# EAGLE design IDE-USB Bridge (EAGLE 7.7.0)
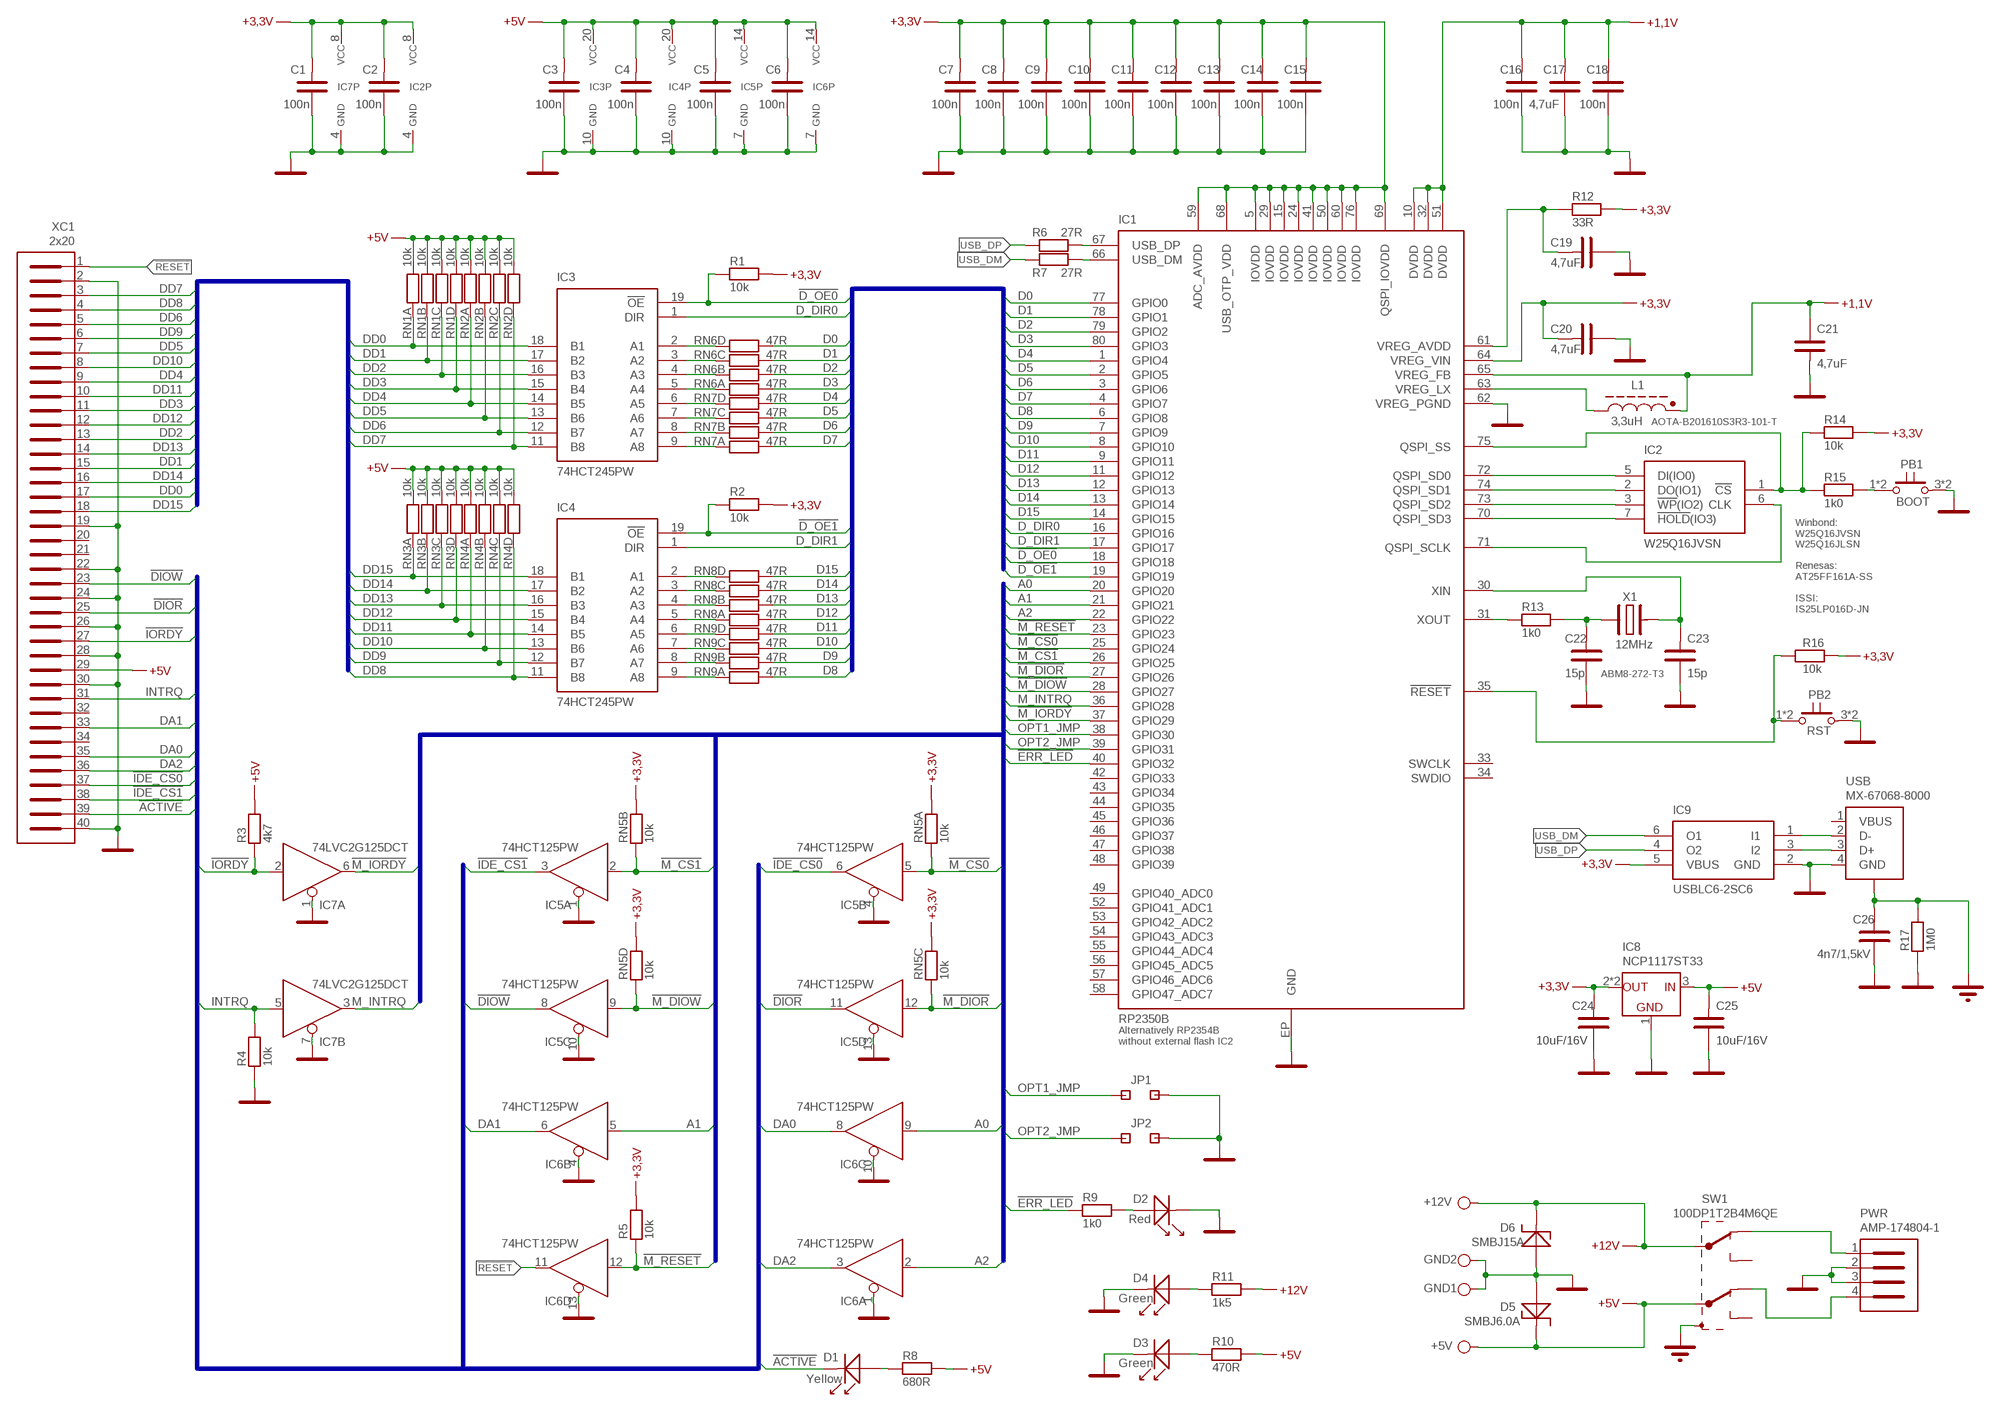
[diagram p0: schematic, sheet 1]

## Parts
+5V  +5V  PAJ_B_16  [P_BOD_16]
+12V  +12V  PAJ_B_16  [P_BOD_16]
C1  100n  CK-SMD-0603  [CK-0603]
C2  100n  CK-SMD-0603  [CK-0603]
C3  100n  CK-SMD-0603  [CK-0603]
C4  100n  CK-SMD-0603  [CK-0603]
C5  100n  CK-SMD-0603  [CK-0603]
C6  100n  CK-SMD-0603  [CK-0603]
C7  100n  CK-SMD-0603  [CK-0603]
C8  100n  CK-SMD-0603  [CK-0603]
C9  100n  CK-SMD-0603  [CK-0603]
C10  100n  CK-SMD-0603  [CK-0603]
C11  100n  CK-SMD-0603  [CK-0603]
C12  100n  CK-SMD-0603  [CK-0603]
C13  100n  CK-SMD-0603  [CK-0603]
C14  100n  CK-SMD-0603  [CK-0603]
C15  100n  CK-SMD-0603  [CK-0603]
C16  100n  CK-SMD-0603  [CK-0603]
C17  4,7uF  CK-SMD-0603  [CK-0603]
C18  100n  CK-SMD-0603  [CK-0603]
C19  4,7uF  CK-SMD-0603  [CK-0603]
C20  4,7uF  CK-SMD-0603  [CK-0603]
C21  4,7uF  CK-SMD-0603  [CK-0603]
C22  15p  CK-SMD-0805  [CK-0805]
C23  15p  CK-SMD-0805  [CK-0805]
C24  10uF/16V  CK-SMD-1206  [CK-1206]
C25  10uF/16V  CK-SMD-1206  [CK-1206]
C26  4n7/1,5kV  CK-SMD-1206  [CK-1206]
D1  Yellow  LED-1206  [LED1206K]
D2  Red  LED-1206  [LED1206K]
D3  Green  LED-1206  [LED1206K]
D4  Green  LED-1206  [LED1206K]
D5  SMBJ6.0A  600W-USM  [DO-214AA]
D6  SMBJ15A  600W-USM  [DO-214AA]
GND1  GND  PAJ_B_16  [P_BOD_16]
GND2  GND  PAJ_B_16  [P_BOD_16]
IC1  RP2350B  RP2350  [QFN80]
IC2  W25Q16JVSN  W25Q16-SN  [SO8]
IC3  74HCT245PW  74245-PW  [TSSOP20]
IC4  74HCT245PW  74245-PW  [TSSOP20]
IC5  74HCT125PW  74125-DT  [TSSOP14]
IC6  74HCT125PW  74125-DT  [TSSOP14]
IC7  74LVC2G125DCT  742G125-DP  [SSOP8]
IC8  NCP1117ST33  LDL1117  [SOT223]
IC9  USBLC6-2SC6  [SOT23-6]
JP1  JMP2-1  [JMP2-1]
JP2  JMP2-1  [JMP2-1]
L1  3,3uH  TL-SMD-2016  [TL-2016]
PB1  BOOT  TL-SMD-PTS647  [TL-PTS647]
PB2  RST  TL-SMD-PTS647  [TL-PTS647]
PWR  AMP-174804-1  AMP174804  [AMP174804]
R1  10k  R-SMD-0805  [R-0805]
R2  10k  R-SMD-0805  [R-0805]
R3  4k7  R-SMD-0805  [R-0805]
R4  10k  R-SMD-0805  [R-0805]
R5  10k  R-SMD-0805  [R-0805]
R6  27R  R-SMD-0805  [R-0805]
R7  27R  R-SMD-0805  [R-0805]
R8  680R  R-SMD-1206  [R-1206]
R9  1k0  R-SMD-1206  [R-1206]
R10  470R  R-SMD-1206  [R-1206]
R11  1k5  R-SMD-1206  [R-1206]
R12  33R  R-SMD-0805  [R-0805]
R13  1k0  R-SMD-0805  [R-0805]
R14  10k  R-SMD-0805  [R-0805]
R15  1k0  R-SMD-0805  [R-0805]
R16  10k  R-SMD-0805  [R-0805]
R17  1M0  R-SMD-1206  [R-1206]
RN1  10k  R-NET4SB  [R-NET4SB]
RN2  10k  R-NET4SB  [R-NET4SB]
RN3  10k  R-NET4SB  [R-NET4SB]
RN4  10k  R-NET4SB  [R-NET4SB]
RN5  10k  R-NET4SB  [R-NET4SB]
RN6  47R  R-NET4SB  [R-NET4SB]
RN7  47R  R-NET4SB  [R-NET4SB]
RN8  47R  R-NET4SB  [R-NET4SB]
RN9  47R  R-NET4SB  [R-NET4SB]
SW1  100DP1T2B4M6QE  SW-100DP1T2B  [SW-100DP1T2]
USB  MX-67068-8000  USB-B-B1  [USB-B1]
X1  12MHz  XTAL-SMD-3225  [X-3225-2]
XC1  2x20  25-V2R40-TOP  [25-V2R40T]

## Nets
!ACTIVE: D1.K XC1.39
!D_OE0: IC1.18(GPIO18) IC3.19(!OE) R1.1
!D_OE1: IC1.19(GPIO19) IC4.19(!OE) R2.1
!DIOR: IC5.11(D:O) XC1.25
!DIOW: IC5.8(C:O) XC1.23
!ERR_LED: IC1.40(GPIO32) R9.1
!IDE_CS0: IC5.6(B:O) XC1.37
!IDE_CS1: IC5.3(A:O) XC1.38
!IORDY: IC7.2(A:I) R3.1 XC1.27
!M_CS0: IC1.25(GPIO24) IC5.5(B:I) RN5.1
!M_CS1: IC1.26(GPIO25) IC5.2(A:I) RN5.2
!M_DIOR: IC1.27(GPIO26) IC5.12(D:I) RN5.3
!M_DIOW: IC1.28(GPIO27) IC5.9(C:I) RN5.4
!M_IORDY: IC1.37(GPIO29) IC7.6(A:O)
!M_RESET: IC1.23(GPIO23) IC6.12(D:I) R5.1
!RESET: IC6.11(D:O) XC1.1
+1,1V: C16.2 C17.2 C18.2 C21.1 IC1.10(DVDD10) IC1.32(DVDD32) IC1.51(DVDD51) IC1.65(VREG_FB) L1.2(K)
+3,3V: C1.2 C2.2 C7.2 C8.2 C9.2 C10.2 C11.2 C12.2 C13.2 C14.2 C15.2 C20.2 C24.2 IC1.5(IOVDD5) IC1.15(IOVDD15) IC1.24(IOVDD24) IC1.29(IOVDD29) IC1.41(IOVDD41) IC1.50(IOVDD50) IC1.59(ADC_AVDD) IC1.60(IOVDD60) IC1.64(VREG_VIN) IC1.68(USB_OTP_VDD) IC1.69(QSPI_IOVDD) IC1.76(IOVDD76) IC2.8(VCC) IC7.8(P:VCC) IC8.2(OUT) IC8.4(OUT) IC9.5(VBUS) R1.2 R2.2 R5.2 R12.2 R14.2 R16.2 RN5.A RN5.B RN5.C RN5.D
+5V: +5V.1 C3.2 C4.2 C5.2 C6.2 C25.2 D5.K IC3.20(VCC) IC4.20(VCC) IC5.14(P:VCC) IC6.14(P:VCC) IC8.3(IN) R3.2 R8.2 R10.2 RN1.A RN1.B RN1.C RN1.D RN2.A RN2.B RN2.C RN2.D RN3.A RN3.B RN3.C RN3.D RN4.A RN4.B RN4.C RN4.D SW1.5 XC1.29
+12V: +12V.1 D6.K R11.2 SW1.2
A0: IC1.20(GPIO20) IC6.9(C:I)
A1: IC1.21(GPIO21) IC6.5(B:I)
A2: IC1.22(GPIO22) IC6.2(A:I)
D0: IC1.77(GPIO0) RN6.D
D1: IC1.78(GPIO1) RN6.C
D2: IC1.79(GPIO2) RN6.B
D3: IC1.80(GPIO3) RN6.A
D4: IC1.1(GPIO4) RN7.D
D5: IC1.2(GPIO5) RN7.C
D6: IC1.3(GPIO6) RN7.B
D7: IC1.4(GPIO7) RN7.A
D8: IC1.6(GPIO8) RN9.A
D9: IC1.7(GPIO9) RN9.B
D10: IC1.8(GPIO10) RN9.C
D11: IC1.9(GPIO11) RN9.D
D12: IC1.11(GPIO12) RN8.A
D13: IC1.12(GPIO13) RN8.B
D14: IC1.13(GPIO14) RN8.C
D15: IC1.14(GPIO15) RN8.D
D_DIR0: IC1.16(GPIO16) IC3.1(DIR)
D_DIR1: IC1.17(GPIO17) IC4.1(DIR)
DA0: IC6.8(C:O) XC1.35
DA1: IC6.6(B:O) XC1.33
DA2: IC6.3(A:O) XC1.36
DD0: IC3.18(B1) RN1.1 XC1.17
DD1: IC3.17(B2) RN1.2 XC1.15
DD2: IC3.16(B3) RN1.3 XC1.13
DD3: IC3.15(B4) RN1.4 XC1.11
DD4: IC3.14(B5) RN2.1 XC1.9
DD5: IC3.13(B6) RN2.2 XC1.7
DD6: IC3.12(B7) RN2.3 XC1.5
DD7: IC3.11(B8) RN2.4 XC1.3
DD8: IC4.11(B8) RN4.4 XC1.4
DD9: IC4.12(B7) RN4.3 XC1.6
DD10: IC4.13(B6) RN4.2 XC1.8
DD11: IC4.14(B5) RN4.1 XC1.10
DD12: IC4.15(B4) RN3.4 XC1.12
DD13: IC4.16(B3) RN3.3 XC1.14
DD14: IC4.17(B2) RN3.2 XC1.16
DD15: IC4.18(B1) RN3.1 XC1.18
GND: C1.1 C2.1 C3.1 C4.1 C5.1 C6.1 C7.1 C8.1 C9.1 C10.1 C11.1 C12.1 C13.1 C14.1 C15.1 C16.1 C17.1 C18.1 C19.1 C20.1 C21.2 C22.1 C23.1 C24.1 C25.1 C26.1 D2.K D3.K D4.K D5.A D6.A GND1.1 GND2.1 IC1.62(VREG_PGND) IC1.EP(GND) IC2.4(GND) IC3.10(GND) IC4.10(GND) IC5.1(A:OE) IC5.4(B:OE) IC5.7(P:GND) IC5.10(C:OE) IC5.13(D:OE) IC6.1(A:OE) IC6.4(B:OE) IC6.7(P:GND) IC6.10(C:OE) IC6.13(D:OE) IC7.1(A:OE) IC7.4(P:GND) IC7.7(B:OE) IC8.1(GND) IC9.2(GND) JP1.2 JP2.2 PB1.3 PB1.4 PB2.3 PB2.4 PWR.2 PWR.3 R4.1 R17.1 USB.4(GND) XC1.2 XC1.19 XC1.22 XC1.24 XC1.26 XC1.28 XC1.30 XC1.40
INTRQ: IC7.5(B:I) R4.2 XC1.31
M_INTRQ: IC1.36(GPIO28) IC7.3(B:O)
N$1: IC1.67(USB_DP) R6.2
N$2: IC1.66(USB_DM) R7.2
N$3: IC1.72(QSPI_SD0) IC2.5(DI(IO0))
N$4: IC1.74(QSPI_SD1) IC2.2(DO(IO1))
N$5: IC1.73(QSPI_SD2) IC2.3(!WP!(IO2))
N$6: IC1.70(QSPI_SD3) IC2.7(!HOLD!(IO3))
N$7: IC1.71(QSPI_SCLK) IC2.6(CLK)
N$8: PB1.1 PB1.2 R15.2
N$9: IC1.75(QSPI_SS) IC2.1(!CS) R14.1 R15.1
N$10: IC1.31(XOUT) R13.1
N$11: C22.2 R13.2 X1.1
N$12: C23.2 IC1.30(XIN) X1.3
N$13: IC1.63(VREG_LX) L1.1(Z)
N$14: IC9.1(I1) USB.2(D-)
N$15: C19.2 IC1.61(VREG_AVDD) R12.1
N$16: IC9.3(I2) USB.3(D+)
N$17: IC3.5(A4) RN6.1
N$18: D3.A R10.1
N$19: D2.A R9.2
N$20: D4.A R11.1
N$21: D1.A R8.1
N$24: IC3.4(A3) RN6.2
N$25: IC3.3(A2) RN6.3
N$26: IC3.2(A1) RN6.4
N$27: IC3.9(A8) RN7.1
N$28: IC3.8(A7) RN7.2
N$29: IC3.7(A6) RN7.3
N$30: IC3.6(A5) RN7.4
N$31: IC4.5(A4) RN8.1
N$32: IC4.4(A3) RN8.2
N$33: IC4.3(A2) RN8.3
N$34: IC4.2(A1) RN8.4
N$35: IC4.9(A8) RN9.1
N$36: IC4.8(A7) RN9.2
N$37: IC4.7(A6) RN9.3
N$38: IC4.6(A5) RN9.4
N$39: IC1.35(!RESET) PB2.1 PB2.2 R16.1
N$40: PWR.1 SW1.1
N$41: PWR.4 SW1.4
OPT1_JMP: IC1.38(GPIO30) JP1.1
OPT2_JMP: IC1.39(GPIO31) JP2.1
PE: C26.2 R17.2 SW1.S1(SHLD) SW1.S2(SHLD) USB.S1(S) USB.S2(S)
USB_DM: IC9.6(O1) R7.1
USB_DP: IC9.4(O2) R6.1
Unconnected: IC1.33(SWCLK) IC1.34(SWDIO) IC1.42(GPIO33) IC1.43(GPIO34) IC1.44(GPIO35) IC1.45(GPIO36) IC1.46(GPIO37) IC1.47(GPIO38) IC1.48(GPIO39) IC1.49(GPIO40_ADC0) IC1.52(GPIO41_ADC1) IC1.53(GPIO42_ADC2) IC1.54(GPIO43_ADC3) IC1.55(GPIO44_ADC4) IC1.56(GPIO45_ADC5) IC1.57(GPIO46_ADC6) IC1.58(GPIO47_ADC7) SW1.3 SW1.6 USB.1(VBUS) XC1.20 XC1.21 XC1.32 XC1.34

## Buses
BUS1:D0,D1,D2,D3,D4,D5,D6,D7,D8,D9,D10,D11,D12,D13,D14,D15,D_DIR0,D_DIR1,!D_OE0,!D_OE1
BUS2:DD0,DD1,DD2,DD3,DD4,DD5,DD6,DD7,DD8,DD9,DD10,DD11,DD12,DD13,DD14,DD15
BUS3:!DIOW,!DIOR,!IORDY,INTRQ,DA1,DA0,DA2,!IDE_CS0,!IDE_CS1,!ACTIVE
BUS4:A0,A1,A2,!M_RESET,!M_CS0,!M_CS1,!M_DIOR,!M_DIOW,M_INTRQ,!M_IORDY,OPT1_JMP,OPT2_JMP,!ERR_LED

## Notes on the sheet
- AOTA-B201610S3R3-101-T
- Winbond:
  W25Q16JVSN
  W25Q16JLSN
  
  Renesas:
  AT25FF161A-SS
  
  ISSI:
  IS25LP016D-JN
- ABM8-272-T3
- Alternatively RP2354B
  without external flash IC2

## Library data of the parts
+5V +12V GND1 GND2 = KONSTR:PAJ_B_16
C1-C26 = PASIV:CK-SMD: SMD keramické vícevrstvé kondenzátory
D1-D4 = DISKRET:LED-1206
D5 D6 = DISKRET:600W-USM
IC1 = INTEL:RP2350
IC2 = MEMORY:W25Q16
IC3 IC4 = IC:74245
IC5 IC6 = 74499:74125
IC7 = 74499:742G125
IC8 = IC:LDL1117: LDO, fixed voltage, input 18V max., 1,2A, high PSRR, ST
IC9 = DISKRET:USBLC6-2
JP1 JP2 = KONSTR:JMP2-1
L1 = PASIV:TL-SMD
PB1 PB2 = KONSTR:TL-SMD
PWR = CONNEC:AMP174804
R1-R17 = PASIV:R-SMD: SMD rezistory
RN1-RN9 = PASIV:R-NET4SB
SW1 = KONSTR:SW-100DP1T2B
USB = CONNEC:USB-B
X1 = PASIV:XTAL-SMD
XC1 = CONNEC:25-V2R40

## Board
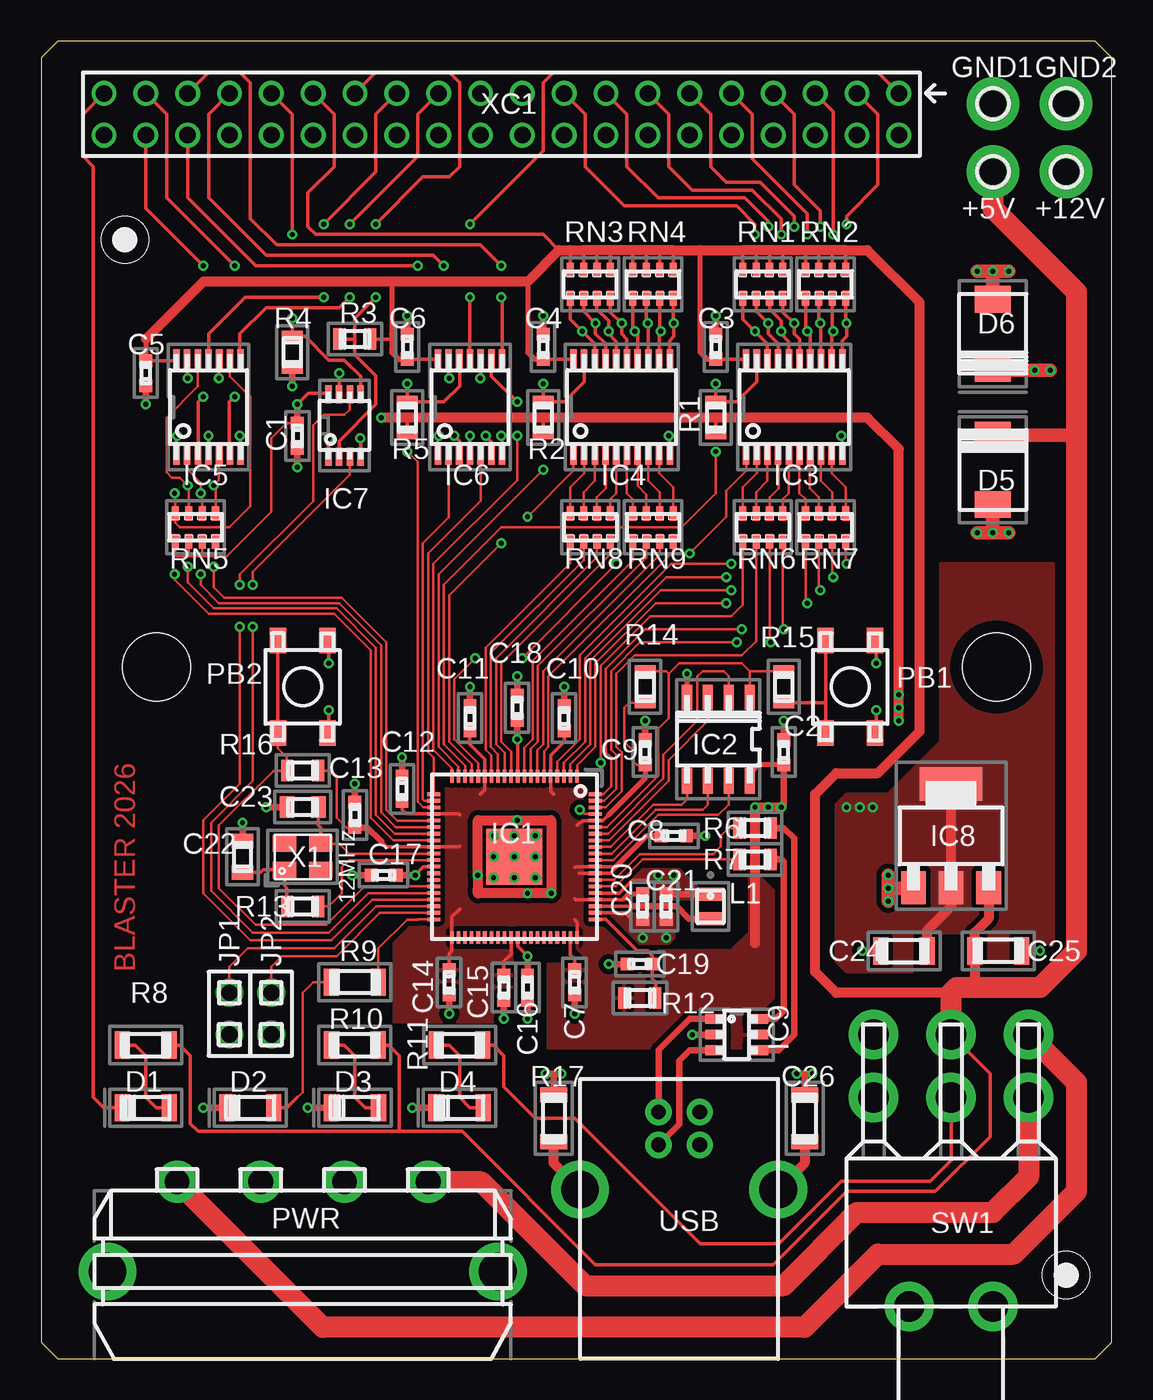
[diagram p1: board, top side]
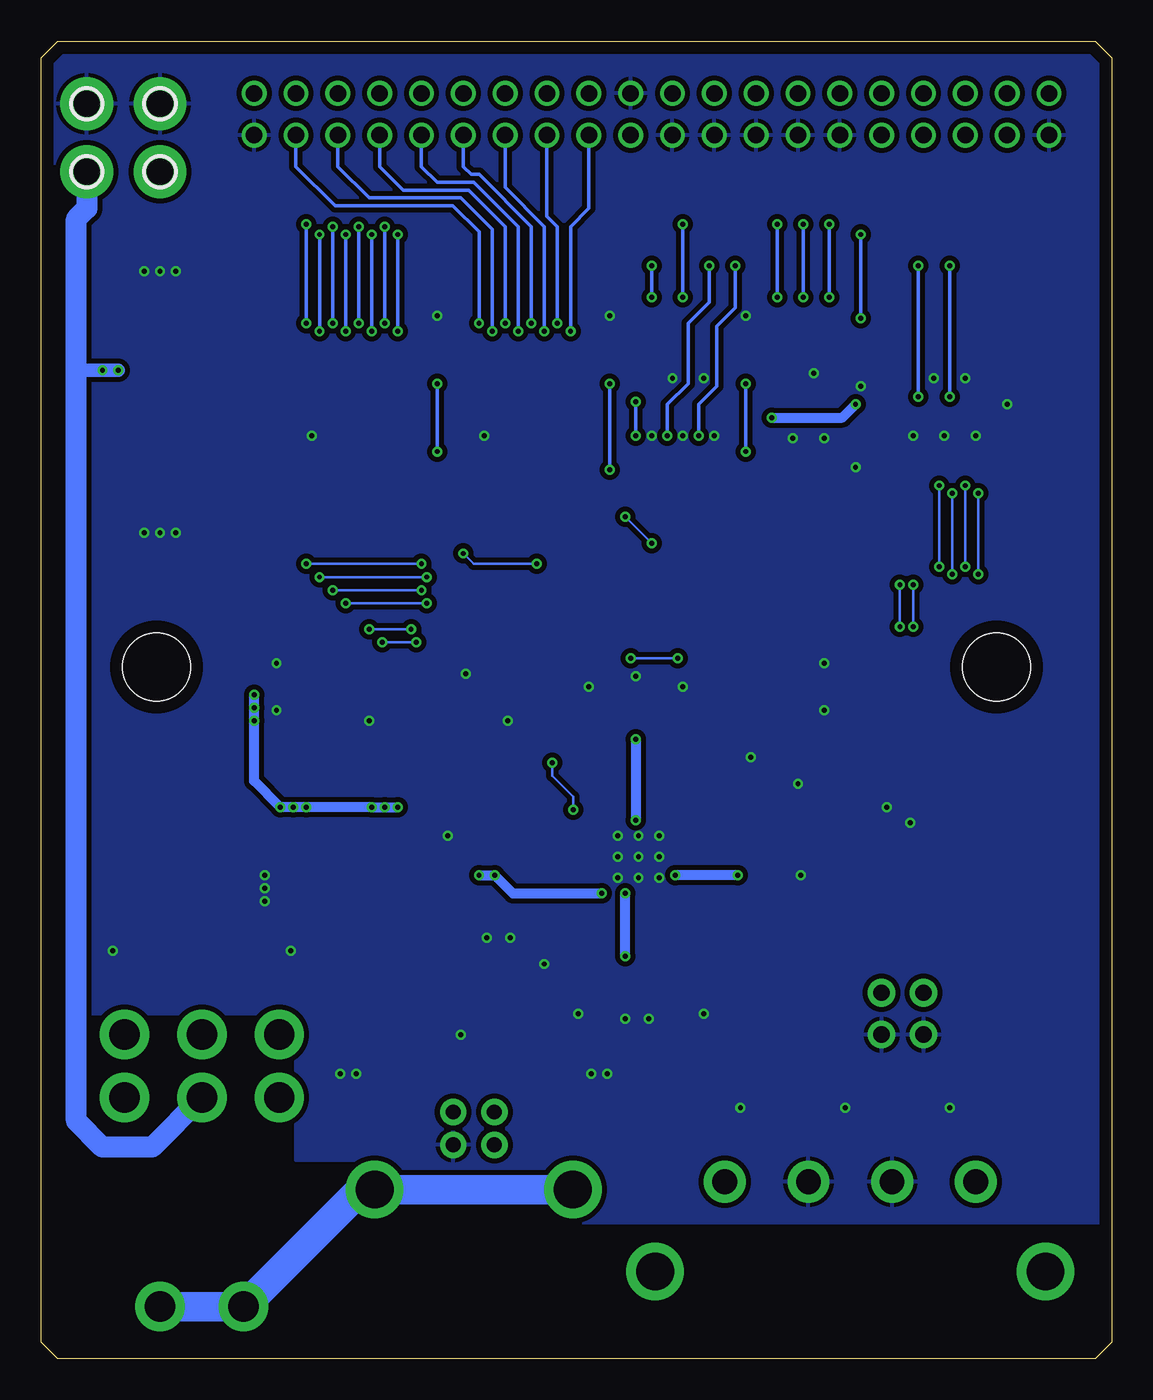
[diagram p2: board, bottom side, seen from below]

Size 65 x 80 mm. Coordinates in mm from the lower left corner, seen from the top.
Outline: 1,0 64,0 65,1 65,79 64,80 1,80 0,79 0,1 1,0
Copper layers (1*16): Top 0.035mm / dielectric 1.5mm / Bottom 0.035mm
Design rules "default *": minimum track width 6mil, minimum drill 10mil, track to track 6mil, track to pad 6mil, pad to pad 6mil, via to via 6mil, smd to smd 6mil, copper to edge 30mil, drill to drill 8mil, minimum pad ring 10mil, minimum via ring 6mil, stop-mask expansion 4mil, vias tented up to drill 15mil, thermal gap 10mil
Holes 4.1 mm at 7,42 58,42

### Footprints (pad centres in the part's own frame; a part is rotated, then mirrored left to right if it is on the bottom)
P_BOD_16 = drill 1.6 pad 3.2: 1 0,0
CK-0603 = smd 0.787 x 0.787: 1 -0.762,0; 2 0.762,0
CK-0805 = smd 0.889 x 1.295: 1 -0.953,0; 2 0.953,0
CK-1206 = smd 0.914 x 1.651: 1 -1.422,0; 2 1.422,0
LED1206K = smd 0.914 x 1.651: A 1.429,0; K -1.429,0
DO-214AA = smd 1.626 x 2.184: A 2.108,0; K -2.108,0
QFN80 = smd 0.78 x 0.22: 1 -4.896,3.8; 2 -4.896,3.4; 3 -4.896,3; 4 -4.896,2.6; 5 -4.896,2.2; 6 -4.896,1.8; 7 -4.896,1.4; 8 -4.896,1; 9 -4.896,0.6; 10 -4.896,0.2; 11 -4.896,-0.2; 12 -4.896,-0.6; 13 -4.896,-1; 14 -4.896,-1.4; 15 -4.896,-1.8; 16 -4.896,-2.2; 17 -4.896,-2.6; 18 -4.896,-3; 19 -4.896,-3.4; 20 -4.896,-3.8; 41 4.896,-3.8; 42 4.896,-3.4; 43 4.896,-3; 44 4.896,-2.6; 45 4.896,-2.2; 46 4.896,-1.8; 47 4.896,-1.4; 48 4.896,-1; 49 4.896,-0.6; 50 4.896,-0.2; 51 4.896,0.2; 52 4.896,0.6; 53 4.896,1; 54 4.896,1.4; 55 4.896,1.8; 56 4.896,2.2; 57 4.896,2.6; 58 4.896,3; 59 4.896,3.4; 60 4.896,3.8 | smd 0.22 x 0.78: 21 -3.8,-4.896; 22 -3.4,-4.896; 23 -3,-4.896; 24 -2.6,-4.896; 25 -2.2,-4.896; 26 -1.8,-4.896; 27 -1.4,-4.896; 28 -1,-4.896; 29 -0.6,-4.896; 30 -0.2,-4.896; 31 0.2,-4.896; 32 0.6,-4.896; 33 1,-4.896; 34 1.4,-4.896; 35 1.8,-4.896; 36 2.2,-4.896; 37 2.6,-4.896; 38 3,-4.896; 39 3.4,-4.896; 40 3.8,-4.896; 61 3.8,4.896; 62 3.4,4.896; 63 3,4.896; 64 2.6,4.896; 65 2.2,4.896; 66 1.8,4.896; 67 1.4,4.896; 68 1,4.896; 69 0.6,4.896; 70 0.2,4.896; 71 -0.2,4.896; 72 -0.6,4.896; 73 -1,4.896; 74 -1.4,4.896; 75 -1.8,4.896; 76 -2.2,4.896; 77 -2.6,4.896; 78 -3,4.896; 79 -3.4,4.896; 80 -3.8,4.896 | smd 3.4 x 3.4: EP 0,0
SO8 = smd 0.61 x 1.524: 1 -1.905,-2.54; 2 -0.635,-2.54; 3 0.635,-2.54; 4 1.905,-2.54; 5 1.905,2.54; 6 0.635,2.54; 7 -0.635,2.54; 8 -1.905,2.54
TSSOP20 = smd 0.4 x 1.2: 1 -2.925,-2.9; 2 -2.275,-2.9; 3 -1.625,-2.9; 4 -0.975,-2.9; 5 -0.325,-2.9; 6 0.325,-2.9; 7 0.975,-2.9; 8 1.625,-2.9; 9 2.275,-2.9; 10 2.925,-2.9; 11 2.925,2.9; 12 2.275,2.9; 13 1.625,2.9; 14 0.975,2.9; 15 0.325,2.9; 16 -0.325,2.9; 17 -0.975,2.9; 18 -1.625,2.9; 19 -2.275,2.9; 20 -2.925,2.9
TSSOP14 = smd 0.4 x 1.2: 1 -1.95,-2.9; 2 -1.3,-2.9; 3 -0.65,-2.9; 4 0,-2.9; 5 0.65,-2.9; 6 1.3,-2.9; 7 1.95,-2.9; 8 1.95,2.9; 9 1.3,2.9; 10 0.65,2.9; 11 0,2.9; 12 -0.65,2.9; 13 -1.3,2.9; 14 -1.95,2.9
SSOP8 = smd 0.4 x 1.1: 1 -0.975,-1.9; 2 -0.325,-1.9; 3 0.325,-1.9; 4 0.975,-1.9; 5 0.975,1.9; 6 0.325,1.9; 7 -0.325,1.9; 8 -0.975,1.9
SOT223 = smd 1.499 x 2.007: 1 -2.286,-3.15; 2 0,-3.15; 3 2.286,-3.15 | smd 3.81 x 2.007: 4 0,3.15
SOT23-6 = smd 0.584 x 1.27: 1 0.953,1.27; 2 0,1.27; 3 -0.953,1.27; 4 -0.953,-1.27; 5 0,-1.27; 6 0.953,-1.27
JMP2-1 = drill 1 pad 1.676: 1 0,0; 2 2.54,0
TL-2016 = smd 0.8 x 1.6: 1 -0.75,0; 2 0.75,0
TL-PTS647 = smd 1.55 x 1: 1 -2.8,1.5; 2 2.8,1.5; 3 -2.8,-1.5; 4 2.8,-1.5
AMP174804 = drill 1.5 pad 2.54: 1 -7.62,0; 2 -2.54,0; 3 2.54,0; 4 7.62,0 | drill 2.3 pad 3.5: S1 -11.85,5.45; S2 11.85,5.45
R-0805 = smd 0.711 x 1.295: 1 -0.953,0; 2 0.953,0
R-1206 = smd 0.914 x 1.651: 1 -1.422,0; 2 1.422,0
R-NET4SB = smd 0.432 x 0.889: 1 -1.219,-0.851; 2 -0.406,-0.851; 3 0.406,-0.851; 4 1.219,-0.851; A -1.219,0.851; B -0.406,0.851; C 0.406,0.851; D 1.219,0.851
SW-100DP1T2 = drill 1.85 pad 3: 1 0,-4.7; 2 0,0; 3 0,4.7; 4 3.81,-4.7; 5 3.81,0; 6 3.81,4.7; S1 -12.7,-2.54; S2 -12.7,2.54
USB-B1 = drill 0.9 pad 1.6: 1 1.25,4.71; 2 -1.25,4.71; 3 -1.25,2.71; 4 1.25,2.71 | drill 2.3 pad 3.5: S1 -6.02,0; S2 6.02,0
X-3225-2 = smd 1.4 x 1: 1 -1.1,-0.8; 2 1.1,-0.8; 3 1.1,0.8; 4 -1.1,0.8
25-V2R40T = drill 1 pad 1.499: 1 0,0; 2 0,2.54; 3 2.54,0; 4 2.54,2.54; 5 5.08,0; 6 5.08,2.54; 7 7.62,0; 8 7.62,2.54; 9 10.16,0; 10 10.16,2.54; 11 12.7,0; 12 12.7,2.54; 13 15.24,0; 14 15.24,2.54; 15 17.78,0; 16 17.78,2.54; 17 20.32,0; 18 20.32,2.54; 19 22.86,0; 20 22.86,2.54; 21 25.4,0; 22 25.4,2.54; 23 27.94,0; 24 27.94,2.54; 25 30.48,0; 26 30.48,2.54; 27 33.02,0; 28 33.02,2.54; 29 35.56,0; 30 35.56,2.54; 31 38.1,0; 32 38.1,2.54; 33 40.64,0; 34 40.64,2.54; 35 43.18,0; 36 43.18,2.54; 37 45.72,0; 38 45.72,2.54; 39 48.26,0; 40 48.26,2.54

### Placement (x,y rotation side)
+5V  57.78,72.07 0 top
+12V  62.23,72.07 0 top
C1  15.56,56.04 90 top
C2  45.09,36.83 270 top
C3  40.96,61.44 270 top
C4  30.48,61.44 270 top
C5  6.35,59.85 90 top
C6  22.23,61.44 270 top
C7  32.38,22.86 90 top
C8  38.42,31.75 180 top
C9  36.67,36.83 270 top
C10  31.75,38.89 270 top
C11  26.04,38.89 270 top
C12  21.91,34.61 270 top
C13  19.05,33.02 270 top
C14  24.77,22.86 90 top
C15  28.1,22.54 90 top
C16  29.53,22.54 90 top
C17  20.8,29.37 0 top
C18  28.89,39.53 270 top
C19  36.35,23.97 0 top
C20  36.51,27.46 90 top
C21  37.94,27.46 270 top
C22  12.22,30.48 270 top
C23  15.88,33.5 0 top
C24  52.39,24.77 0 top
C25  58.1,24.77 180 top
C26  46.35,14.61 270 top
D1  6.35,15.24 0 top
D2  12.7,15.24 0 top
D3  19.05,15.24 0 top
D4  25.4,15.24 0 top
D5  57.78,53.98 270 top
D6  57.78,62.23 90 top
GND1  57.78,76.2 0 top
GND2  62.23,76.2 0 top
IC1  28.73,30.48 270 top
IC2  41.12,37.62 180 top
IC3  45.72,57.78 0 top
IC4  35.24,57.78 0 top
IC5  10.16,57.78 0 top
IC6  26.04,57.78 0 top
IC7  18.41,56.67 0 top
IC8  55.24,31.75 0 top
IC9  42.23,19.68 90 top
JP1  11.43,22.23 270 top
JP2  13.97,22.23 270 top
L1  40.64,27.46 90 top
PB1  49.12,40.8 90 top
PB2  15.88,40.8 90 top
PWR  15.88,10.75 180 top
R1  40.96,57.15 270 top
R2  30.48,57.15 270 top
R3  19.05,61.91 0 top
R4  15.24,61.12 90 top
R5  22.23,57.15 270 top
R6  43.34,32.23 180 top
R7  43.34,30.32 180 top
R8  6.35,19.05 0 top
R9  19.05,22.86 180 top
R10  19.05,19.05 0 top
R11  25.4,19.05 0 top
R12  36.35,21.91 180 top
R13  15.88,27.46 180 top
R14  36.67,40.8 270 top
R15  45.09,40.8 270 top
R16  15.88,35.72 0 top
R17  31.11,14.61 270 top
REF1  [REF-K]  5.08,67.94 0 top
REF2  [REF-K]  62.23,5.08 0 top
RN1  43.81,65.25 0 top
RN2  47.62,65.25 0 top
RN3  33.34,65.25 0 top
RN4  37.15,65.25 0 top
RN5  9.37,50.48 180 top
RN6  43.81,50.48 180 top
RN7  47.62,50.48 180 top
RN8  33.34,50.48 180 top
RN9  37.15,50.48 180 top
SW1  55.24,15.88 90 top
USB  38.73,10.28 0 top
X1  15.88,30.48 0 top
XC1  52.07,76.83 180 top

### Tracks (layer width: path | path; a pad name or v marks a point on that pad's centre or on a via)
!ACTIVE
  Top 0.203: XC1.39 2.54,75.56 2.54,73.03 3.17,72.39 3.17,15.88 3.81,15.24 D1.K
!D_OE0  (via drill 0.3)
  Top 0.152: IC1.18 25.73,36.02 24.45,37.31 24.45,46.99 27.94,50.48 38.89,50.48 40.96,52.55 v40.96,55.09
  Top 0.203: IC3.19 43.45,59.32 42.23,58.1 R1.1 v40.96,59.21
  Bottom 0.203: v40.96,59.21 v40.96,55.09
!D_OE1  (via drill 0.3)
  Top 0.152: IC1.19 25.33,35.94 24.13,37.15 24.13,47.62 v30.48,53.98
  Top 0.203: IC4.19 32.97,59.32 31.75,58.1 R2.1 v30.48,59.21
  Bottom 0.203: v30.48,59.21 v30.48,53.98
!DIOR  (via drill 0.3)
  Top 0.203: IC5.11 10.16,62.23 12.38,64.45 v17.14,64.45 | v17.14,68.9 20.32,72.07 20.32,75.56 XC1.25
  Bottom 0.203: v17.14,64.45 v17.14,68.9
!DIOW  (via drill 0.3)
  Top 0.203: IC5.8 12.06,60.69 12.06,62.23 13.65,63.82 18.1,63.82 v18.73,64.45 | XC1.23 22.86,75.56 22.86,73.03 v18.73,68.9
  Bottom 0.203: v18.73,64.45 v18.73,68.9
!ERR_LED
  Top 0.152: IC1.40 22.87,26.68 22.86,26.67 22.23,26.67 20.47,24.92 R9.1
!IDE_CS0  (via drill 0.3)
  Top 0.203: XC1.37 7.62,75.56 7.62,70.48 v11.75,66.36 | IC5.6 11.43,54.88 11.43,58.1 v11.75,58.42
  Bottom 0.203: v11.75,58.42 v11.75,66.36
!IDE_CS1  (via drill 0.3)
  Top 0.203: IC5.3 9.53,54.88 9.53,58.1 v9.84,58.42 | XC1.38 6.35,69.85 v9.84,66.36
  Bottom 0.203: v9.84,58.42 v9.84,66.36
!IORDY  (via drill 0.3)
  Top 0.203: IC7.2 18.09,55.71 20.32,57.94 20.32,59.69 19.05,60.96 19.05,61.91 | XC1.27 20.32,78.11 24.77,78.11 25.4,77.47 25.4,72.39 24.77,71.75 23.18,71.75 v20.32,68.9 | v20.32,64.45 19.05,63.18 19.05,61.91 | R3.1 19.05,61.91
  Bottom 0.203: v20.32,68.9 v20.32,64.45
!M_CS0  (via drill 0.3)
  Top 0.152: IC1.25 21.61,32.68 20.95,33.34 20.95,43.5 18.26,46.2 11.11,46.2 10.48,46.83 v10.48,48.1 | RN5.1 10.59,52.91 v10.48,53.02 10.79,53.34 10.79,54.87
  Top 0.203: 10.79,54.87 IC5.5
  Bottom 0.152: v10.48,48.1 v10.48,53.02
!M_CS1  (via drill 0.3)
  Top 0.152: IC1.26 21.54,32.28 20.64,33.18 20.64,43.34 18.1,45.88 10.79,45.88 9.68,46.99 v9.68,47.62 | RN5.2 9.77,52.46 v9.68,52.55 9.68,53.18 8.86,54.01 IC5.2
  Top 0.203: 8.89,54.85 IC5.2
  Bottom 0.152: v9.68,47.62 v9.68,52.55
!M_DIOR  (via drill 0.3)
  Top 0.152: IC1.27 21.46,31.88 20.32,33.02 20.32,43.18 17.94,45.56 10.48,45.56 8.89,47.15 v8.89,48.1 | RN5.3 8.96,52.95 | IC5.12 9.51,59.04 7.62,57.15 7.62,53.82 7.94,53.5 8.41,53.5 v8.89,53.02
  Top 0.203: 8.96,52.95 v8.89,53.02
  Bottom 0.152: v8.89,48.1 v8.89,53.02
!M_DIOW  (via drill 0.3)
  Top 0.152: IC1.28 21.38,31.48 20,32.86 20,43.02 17.78,45.24 10.16,45.24 8.1,47.31 v8.1,47.62 | RN5.4 8.15,52.49 | IC5.9 11.46,59.66 12.7,58.42 12.7,51.75 11.43,50.48 8.41,50.48 8.15,50.75 8.15,51.07
  Top 0.203: 8.15,52.49 v8.1,52.55 | RN5.4 8.15,51.07
  Bottom 0.152: v8.1,47.62 v8.1,52.55
!M_IORDY  (via drill 0.3)
  Top 0.152: IC1.37 20.1,27.88 17.62,25.4 12.7,25.4 9.84,28.26 9.84,32.7 12.06,34.92 v12.06,44.45 | IC7.6 18.74,57.63 18.41,57.31 17.14,57.31 16.51,56.67 16.51,52.07 12.06,47.62 v12.06,46.99
  Bottom 0.152: v12.06,46.99 v12.06,44.45
!M_RESET  (via drill 0.3)
  Top 0.152: IC1.23 23.19,33.48 22.86,33.81 22.86,54.45 v22.23,55.09
  Top 0.203: IC6.12 25.4,59.05 24.45,58.1 R5.1 v22.23,59.21
  Bottom 0.203: v22.23,59.21 v22.23,55.09
!RESET  (via drill 0.3)
  Top 0.203: XC1.1 50.8,78.11 31.11,78.11 30.48,77.47 30.48,73.34 v26.04,68.9 | IC6.11 v26.04,64.45
  Bottom 0.203: v26.04,64.45 v26.04,68.9
+1,1V  (via drill 0.3)
  Top 0.203: IC1.65 35.11,28.28 35.88,29.05 36.67,29.05 | IC1.51 28.93,25.04 v29.53,24.45 | IC1.10 28.93,37.58 v28.89,37.62 | IC1.32 23.21,29.88 v22.7,29.37
  Top 0.406: L1.2 37.95,28.21 C21.1 | C16.2 v29.53,24.45 | C18.2 v28.89,37.62 | v22.7,29.37 C17.2
  Top 0.61: v30.96,28.26 v29.53,28.26 26.51,28.26 26.51,28.57 v26.51,29.37 26.51,32.7 v28.89,32.7 30.96,32.7 v30.96,28.26
  Bottom 0.61: v38.42,29.37 v37.47,29.37 36.35,28.26 v30.96,28.26 | v29.53,24.45 v29.53,28.26 | v28.89,37.62 v28.89,32.7 | v22.7,29.37 v26.51,29.37
  pour Top (no thermals): 35.88,29.05 37.31,29.05 37.31,27.94 40.01,27.94 40.01,28.42 38.73,29.69 36.51,29.69
+3,3V  (via drill 0.3)
  Top 0.152: R14.2 35.72,39.85 35.4,39.53 35.4,37.47 35.88,36.99 35.88,36.35 36.16,36.07 C9.2 | R16.2 17.46,35.72 17.94,35.24 17.94,32.86 18.54,32.26 C13.2 | RN5.D 8.15,48.74 8.96,48.74 | RN5.C 8.96,48.74 | 8.96,48.74 9.77,48.74 | RN5.B 9.77,48.74 | 9.77,48.74 10.59,48.74 | 10.59,48.74 RN5.A | 10.59,48.74 11.27,48.74 13.97,51.44 13.97,55.88 14.89,56.8 C1.2
  Top 0.203: 34.45,33.02 34.11,32.68 IC1.76 32.84,32.68 32.54,32.38 | C10.2 31.75,37.47 30.93,36.65 IC1.5 30.93,34.47 31.11,34.29 | C11.2 26.04,37.31 26.93,36.41 IC1.15 26.93,34.55 26.67,34.29 | C12.2 21.91,33.34 22.16,33.08 IC1.24 25.34,33.08 25.4,33.02 | 20.64,31.43 20.99,31.08 IC1.29 25.36,31.08 25.4,31.11 | IC1.59 32.13,24.54 32.38,24.29 C7.2 | C14.2 24.77,24.61 24.93,24.77 IC1.41 24.93,26.84 25.4,27.3 | C15.2 28.1,24.13 28.53,24.57 IC1.50 | IC1.60 32.53,26.52 32.38,26.67 | 32.38,27.94 32.45,27.88 IC1.64 35.34,27.88 35.48,28.02 | 32.38,29.84 32.42,29.88 IC1.69 34.89,29.88 34.92,29.84 34.56,29.48 IC1.68 | 32.66,29.48 33.38,29.48 | R1.2 40.96,56.83 41.27,57.15 | R2.2 30.48,57.15 | R5.2 22.23,57.15 | IC7.8 17.44,58.61 16.22,58.61 v15.56,57.94
  Top 0.305: 35.4,27.94 35.48,28.02 35.69,28.23 C20.2 | C8.2 36.76,31.75 34.89,29.88 | C9.2 36.67,35.24 34.45,33.02 | IC2.8 43.02,35.56 43.53,36.07 C2.2
  Top 0.406: C13.2 19.81,32.26 20.64,31.43 | v44.93,33.5 45.09,33.66 C2.2 | C1.2 v15.56,57.94
  Top 0.61: 43.34,25.24 v43.34,33.5 v44.13,33.5 v44.93,33.5 | C24.2 53.81,26.03 55.24,27.46 IC8.2 IC8.4 | v20.64,57.15 22.23,57.15 30.48,57.15 41.27,57.15 50.16,57.15 52.07,55.24 v52.07,40.32 v52.07,39.53 v52.07,38.73
  Bottom 0.61: v52.07,40.32 v52.07,38.73 52.07,35.08 v50.48,33.5 v44.93,33.5 v44.13,33.5 v43.34,33.5 | v20.64,57.15 16.35,57.15 v15.56,57.94
  other vias: 49.69,33.5 48.9,33.5
  pour Top (isolate 0.305): 35.56,24.77 41.91,24.77 43.02,25.88 43.02,29.21 43.66,29.21 44.45,28.42 44.45,21.91 43.81,21.27 43.81,18.89 30.8,18.89 30.8,23.97 33.02,23.97 33.02,24.45 32.54,24.92 32.54,26.35 27.46,26.35 27.46,24.77 28.57,24.77 28.57,20.48 21.43,20.48 21.43,26.67 24.61,26.67 24.61,34.61 32.86,34.61 32.86,27.46
  pour Top (isolate 0.305, no thermals): 48.26,33.66 48.26,24.13 48.9,23.5 52.86,23.5 52.86,25.88 56.52,25.88 56.52,24.13 60.33,24.13 61.44,25.24 61.44,48.26 54.61,48.26 54.61,37.47 51.44,34.29 48.9,34.29
+5V
  Top 0.203: SW1.5 57.63,17.3 57.63,13.49 54.29,10.16 48.9,10.16 44.45,5.71 33.66,5.71 25.56,13.81 21.75,13.81 | 21.75,13.81 21.75,18.41 21.11,19.05 R10.2 | R8.2 8.41,19.05 9.05,18.41 9.05,14.29 9.53,13.81 21.75,13.81 | RN3.A 32.12,67.31 | 32.93,67.31 RN3.B | RN3.C 33.74,67.31 | RN3.D 34.56,67.31 | RN4.A 35.93,67.31 | RN4.B 36.74,67.31 | RN4.C 37.55,67.31 | RN4.D 38.37,67.31 | RN1.A 42.6,67.31 | RN1.B 43.41,67.31 | RN1.C 44.22,67.31 | RN1.D 45.03,67.31 | RN2.A 46.41,67.31 | RN2.B 47.22,67.31 | RN2.C 48.03,67.31 | RN2.D 48.84,67.31 | 24.09,60.83 IC6.14 C6.2 | C3.2 IC3.20 | C4.2 IC4.20 | R3.2 21.27,61.91 21.27,62.23 | IC5.14 8.21,60.61 C5.2 | XC1.29 17.78,75.56 17.78,72.39 16.19,70.8 16.19,68.74 16.67,68.26 30.48,68.26 31.43,67.31
  Top 0.305: 40.01,67.31 40.01,61.12 40.45,60.67 C3.2 | 29.53,65.41 29.53,61.12 29.97,60.67 C4.2 | 21.27,65.41 21.27,62.23 21.27,61.12 21.72,60.67 C6.2 | 6.35,61.91 C5.2
  Top 0.61: IC8.3 57.53,26.73 56.68,25.88 C25.2 56.68,22.54 56.52,22.54 | 55.24,22.23 48.26,22.23 46.99,23.5 46.99,34.29 48.26,35.56 50.8,35.56 53.34,38.1 53.34,64.14 50.16,67.31 48.84,67.31 48.03,67.31 47.22,67.31 46.41,67.31 45.03,67.31 44.22,67.31 43.41,67.31 42.6,67.31 40.01,67.31 38.37,67.31 37.55,67.31 36.74,67.31 35.93,67.31 34.56,67.31 33.74,67.31 32.93,67.31 32.12,67.31 31.43,67.31 29.53,65.41 21.27,65.41 9.84,65.41 6.35,61.91 | 62.66,56.08 62.87,55.88
  Top 0.813: D5.K 62.66,56.08
  Top 1.27: SW1.5 55.24,22.23 55.56,22.54 56.52,22.54 60.64,22.54 62.87,24.77 62.87,55.88 62.87,64.77 57.78,69.85 +5V.1
+12V  (via drill 0.3)
  Top 0.203: SW1.2 55.24,12.06 53.98,10.79 48.58,10.79 44.77,6.99 40.01,6.99 32.38,14.61 30,14.61 28.1,16.51 28.1,18.41 27.46,19.05 R11.2
  Top 0.61: D6.K 57.78,60.01
  Top 0.813: 57.78,60.01 v60.33,60.01 v61.28,60.01
  Bottom 0.813: 62.87,60.01 v61.28,60.01 v60.33,60.01
  Bottom 1.27: SW1.2 58.26,12.86 61.28,12.86 62.87,14.45 62.87,60.01 62.87,69.22 62.23,69.85 +12V.1
A0  (via drill 0.3)
  Top 0.152: IC1.20 24.93,35.87 23.81,36.99 23.81,48.26 28.89,53.34 v28.89,56.04
  Top 0.203: IC6.9 27.34,59.66 v28.89,58.1
  Bottom 0.203: v28.89,58.1 v28.89,56.04
A1
  Top 0.152: IC1.21 23.84,36.49 23.5,36.83 23.5,48.9 26.68,52.09 IC6.5
A2
  Top 0.152: IC1.22 23.27,33.88 23.18,33.97 23.18,49.53 24.73,51.09 IC6.2
D0  (via drill 0.3)
  Top 0.152: v33.97,36.2 33.97,42.07 36.99,45.09 41.91,45.09 42.6,45.77 RN6.D | IC1.77 32.96,33.08 v32.7,33.34
  Bottom 0.152: v32.7,33.34 32.7,34.13 33.97,35.4 v33.97,36.2
D1
  Top 0.152: IC1.78 34.27,33.48 35.24,34.45 35.24,36.83 34.92,37.15 34.92,41.59 36.04,42.7 42.55,42.7 43.41,43.57 RN6.C
D2  (via drill 0.3)
  Top 0.152: RN6.B 44.22,43.57 | IC1.79 34.2,33.88 34.92,34.61 34.92,36.67 34.61,36.99 34.61,41.75 36.35,43.5 v42.23,43.5
  Top 0.203: v44.29,43.5 44.22,43.57
  Bottom 0.152: v42.23,43.5 v44.29,43.5
D3  (via drill 0.3)
  Top 0.152: v42.55,44.29 36.67,44.29 34.29,41.91 34.29,36.83 34.61,36.51 34.61,34.77 34.12,34.28 IC1.80 | RN6.A 45.03,44.34
  Top 0.203: v45.09,44.29 45.03,44.34
  Bottom 0.152: v42.55,44.29 v45.09,44.29
D4  (via drill 0.3)
  Top 0.152: IC1.1 32.53,36.03 33.66,37.15 33.66,42.23 37.31,45.88 v41.59,45.88 | RN7.D 46.41,45.99 v46.51,45.88
  Bottom 0.152: v41.59,45.88 v46.51,45.88
D5  (via drill 0.3)
  Top 0.152: IC1.2 32.13,36.1 33.34,37.31 33.34,42.39 37.62,46.67 v41.91,46.67 | RN7.C 47.22,46.76 v47.31,46.67
  Bottom 0.152: v41.91,46.67 v47.31,46.67
D6  (via drill 0.3)
  Top 0.152: IC1.3 31.73,36.18 33.02,37.47 33.02,42.55 37.94,47.47 v41.59,47.47 | RN7.B 48.03,47.54 v48.1,47.47
  Bottom 0.152: v41.59,47.47 v48.1,47.47
D7  (via drill 0.3)
  Top 0.152: IC1.4 31.33,36.26 32.7,37.62 32.7,42.7 38.26,48.26 v41.91,48.26 | RN7.A 48.84,48.31 v48.9,48.26
  Bottom 0.152: v41.91,48.26 v48.9,48.26
D8
  Top 0.152: IC1.6 30.53,36.88 30.8,37.15 30.8,41.43 38.37,49 RN9.A
D9
  Top 0.152: IC1.7 30.13,36.96 30.48,37.31 30.48,41.75 37.55,48.83 RN9.B
D10
  Top 0.152: IC1.8 29.73,37.04 30.16,37.47 30.16,42.07 36.74,48.65 RN9.C
D11
  Top 0.152: IC1.9 29.33,37.11 29.84,37.62 29.84,42.39 35.93,48.47 RN9.D
D12
  Top 0.152: IC1.11 28.53,36.87 27.94,37.47 27.94,42.23 34.56,48.84 RN8.A
D13
  Top 0.152: IC1.12 28.13,36.8 27.62,37.31 27.62,42.55 33.74,48.67 RN8.B
D14
  Top 0.152: IC1.13 27.73,36.72 27.3,37.15 27.3,42.86 32.93,48.49 RN8.C
D15
  Top 0.152: IC1.14 27.33,36.64 26.99,36.99 26.99,43.18 32.12,48.31 RN8.D
D_DIR0  (via drill 0.3)
  Top 0.152: IC1.16 26.53,36.17 25.08,37.62 25.08,41.27 v26.35,42.55 | IC3.1 42.8,53.91 41.59,52.7 41.59,51.12 v39.37,48.9 | v29.21,42.55 v34.92,48.26
  Bottom 0.152: v26.35,42.55 v29.21,42.55 | v34.92,48.26 38.73,48.26 v39.37,48.9
D_DIR1  (via drill 0.3)
  Top 0.152: IC1.17 26.13,36.1 24.77,37.47 24.77,46.35 v27.94,49.53 | IC4.1 32.32,53.91 v29.53,51.12
  Bottom 0.152: v27.94,49.53 v29.53,51.12
DA0  (via drill 0.3)
  Top 0.203: IC6.8 27.98,64.41 v27.94,64.45 | XC1.35 10.16,78.11 12.06,78.11 12.7,77.47 12.7,69.22 14.29,67.63 26.67,67.63 v27.94,66.36
  Bottom 0.203: v27.94,64.45 v27.94,66.36
DA1  (via drill 0.3)
  Top 0.203: IC6.6 27.34,55.69 v26.99,56.04 | XC1.33 10.16,75.56 10.16,70.48 13.65,66.99 23.81,66.99 v24.45,66.36
  Bottom 0.203: v26.99,56.04 26.99,57.94 25.72,59.21 25.72,62.87 24.45,64.14 v24.45,66.36
DA2  (via drill 0.3)
  Top 0.203: XC1.36 8.89,70.48 13.02,66.36 v22.86,66.36 | IC6.3 25.39,55.74 v25.08,56.04
  Bottom 0.203: v25.08,56.04 25.08,57.94 23.97,59.05 23.97,62.71 22.86,63.82 v22.86,66.36
DD0  (via drill 0.3)
  Top 0.203: XC1.17 33.02,75.56 33.02,72.39 35.4,70.01 42.23,70.01 43.34,68.9 v43.34,68.26 | IC3.18 44.09,61.63 v43.34,62.39 42.6,63.13 RN1.1
  Bottom 0.203: v43.34,68.26 v43.34,62.39
DD1  (via drill 0.3)
  Top 0.203: XC1.15 35.56,75.56 35.56,72.39 37.47,70.48 42.7,70.48 44.13,69.06 v44.13,68.74 | IC3.17 44.74,61.62 44.13,62.23 v44.13,62.87 43.41,63.59 RN1.2
  Bottom 0.203: v44.13,68.74 v44.13,62.87
DD2  (via drill 0.3)
  Top 0.203: XC1.13 38.1,75.56 38.1,72.39 39.53,70.96 43.18,70.96 44.93,69.22 v44.93,68.26 | RN1.3 44.22,63.73 44.93,63.02 v44.93,62.39 44.93,62.23 45.4,61.75 45.4,60.69 IC3.16
  Bottom 0.203: v44.93,68.26 v44.93,62.39
DD3  (via drill 0.3)
  Top 0.203: XC1.11 40.64,75.56 40.64,72.39 41.59,71.44 43.66,71.44 45.72,69.37 v45.72,68.74 | IC3.15 46.05,61.91 45.72,62.23 v45.72,62.87 45.03,63.55 RN1.4
  Bottom 0.203: v45.72,68.74 v45.72,62.87
DD4  (via drill 0.3)
  Top 0.203: XC1.9 43.18,75.56 43.18,72.87 46.51,69.53 v46.51,68.26 | IC3.14 46.7,62.21 v46.51,62.39 46.41,62.5 RN2.1
  Bottom 0.203: v46.51,68.26 v46.51,62.39
DD5  (via drill 0.3)
  Top 0.203: IC3.13 47.34,62.83 v47.31,62.87 47.22,62.95 RN2.2 | XC1.7 45.72,75.56 45.72,71.28 47.31,69.69 v47.31,68.74
  Bottom 0.203: v47.31,68.74 v47.31,62.87
DD6  (via drill 0.3)
  Top 0.203: XC1.5 48.1,75.72 v48.1,68.26 | IC3.12 47.99,62.28 v48.1,62.39 48.03,62.46 RN2.3
  Bottom 0.203: v48.1,68.26 v48.1,62.39
DD7  (via drill 0.3)
  Top 0.203: XC1.3 50.8,75.56 50.8,71.28 48.9,69.37 v48.9,68.9 | IC3.11 48.65,61.82 48.9,62.07 v48.9,62.87 48.84,62.92 RN2.4
  Bottom 0.203: v48.9,68.9 v48.9,62.87
DD8  (via drill 0.3)
  Top 0.203: RN4.4 38.37,62.92 v38.42,62.87 38.42,62.07 38.17,61.82 IC4.11
  Bottom 0.203: XC1.4 49.53,72.39 47.15,70.01 40.01,70.01 38.42,68.42 v38.42,62.87
DD9  (via drill 0.3)
  Top 0.203: RN4.3 37.55,62.46 v37.62,62.39 37.52,62.28 IC4.12
  Bottom 0.203: XC1.6 46.99,72.39 45.09,70.48 39.53,70.48 37.62,68.58 v37.62,62.39
DD10  (via drill 0.3)
  Top 0.203: RN4.2 36.74,62.95 v36.83,62.87 36.87,62.83 IC4.13
  Bottom 0.203: XC1.8 44.45,72.39 43.02,70.96 39.05,70.96 36.83,68.74 v36.83,62.87
DD11  (via drill 0.3)
  Top 0.203: RN4.1 35.93,62.5 v36.04,62.39 36.22,62.21 IC4.14
  Bottom 0.203: XC1.10 41.91,72.39 40.96,71.44 38.73,71.44 36.04,68.74 v36.04,62.39
DD12  (via drill 0.3)
  Top 0.203: RN3.4 34.56,63.55 v35.24,62.87 35.24,62.23 35.57,61.91 IC4.15
  Bottom 0.203: XC1.12 39.37,72.39 38.89,71.91 38.42,71.91 35.24,68.74 v35.24,62.87
DD13  (via drill 0.3)
  Top 0.203: RN3.3 33.74,63.73 34.45,63.02 v34.45,62.39 34.45,62.23 34.92,61.75 34.92,60.69 IC4.16
  Bottom 0.203: v34.45,62.39 34.45,68.74 36.83,71.12 XC1.14
DD14  (via drill 0.3)
  Top 0.203: RN3.2 32.93,63.59 v33.66,62.87 33.66,62.23 34.27,61.62 IC4.17
  Bottom 0.203: v33.66,62.87 33.66,68.74 34.29,69.37 XC1.16
DD15  (via drill 0.3)
  Top 0.203: RN3.1 32.12,63.13 v32.86,62.39 33.62,61.63 IC4.18
  Bottom 0.203: v32.86,62.39 32.86,68.74 31.75,69.85 XC1.18
GND  (via drill 0.3)
  Top 0.203: v30,31.75 v28.73,31.75 v27.46,31.75 v27.46,30.48 v27.46,29.21 v28.73,29.21 | v30,30.48 v30,29.21 v28.73,29.21 | IC1.EP v28.73,29.21 | IC1.62 35.47,27.08 35.72,26.83 | IC4.10 38.17,55.97 v38.1,56.04 | IC3.10 48.65,55.97 v48.58,56.04 | IC6.7 27.98,55.99 v27.94,56.04 | IC6.4 v26.04,56.04 | IC6.10 26.68,59.55 v26.67,59.53 | IC6.13 24.73,59.56 v24.77,59.53 | IC5.1 8.21,55.99 v8.26,56.04 | IC5.7 12.11,55.99 v12.06,56.04 | IC5.10 10.81,59.55 v10.79,59.53 | IC7.4 19.39,55.86 v19.37,55.88 | IC7.1 17.44,55.86 v17.46,55.88 | IC5.4 v10.16,56.04 | IC5.13 8.86,59.56 v8.89,59.53 | IC6.1 24.09,55.99 v24.13,56.04 | IC7.7 18.1,58.58 v18.1,59.85 | 50.55,38 PB1.3 50.71,38 v50.71,39.37 | 50.55,43.6 PB1.4 50.71,43.6 v50.71,42.23 | 17.3,38 PB2.3 17.46,38 v17.46,39.37 | 17.3,43.6 PB2.4 17.46,43.6 v17.46,42.23
  Top 0.305: IC2.4 v39.21,41.59
  Top 0.406: C19.1 v34.45,23.97 | C2.1 v45.09,38.73 | C9.1 v36.67,38.73 | C8.1 v40.32,31.75 | C10.1 v31.75,40.8 | C18.1 v28.89,41.43 | C11.1 v26.04,40.8 | C12.1 v21.91,36.51 | C13.1 v19.05,34.92 | C22.1 v12.22,32.54 | C23.1 v13.65,33.5 | C17.1 v18.89,29.37 | C7.1 v32.38,20.95 | C16.1 v29.53,20.64 | C15.1 v28.1,20.64 | C14.1 v24.77,20.95 | IC9.2 v39.53,19.68 | v9.84,15.24 D2.K | v16.19,15.24 D3.K | v22.54,15.24 D4.K | v49.85,24.77 C24.1 | v60.64,24.77 C25.1 | C4.1 v30.48,63.34 | C3.1 v40.96,63.34 | C6.1 v22.23,63.34 | C5.1 v6.35,57.94 | C1.1 v15.56,54.13 | R4.1 v15.24,59.05 | v45.88,17.3 46.35,17.3 | 46.35,17.3 v46.83,17.3 | C26.1 46.35,17.3 | v30.64,17.3 31.11,17.3 | 31.11,17.3 v31.59,17.3 | R17.1 31.11,17.3
  Top 0.61: 52.86,28.6 IC8.1 52.96,28.57
  Top 0.813: v51.44,29.37 v51.44,28.57 | v51.44,28.57 v51.44,27.78 | v51.44,28.57 52.96,28.57 | v56.83,66.04 v57.78,66.04 | v57.78,66.04 v58.74,66.04 | D6.A v57.78,66.04 | v56.83,50.16 v57.78,50.16 | v57.78,50.16 v58.74,50.16 | D5.A v57.78,50.16
  other vias: 36.51,25.56 37.94,25.56 28.73,30.48
  pour Top (rank 2, no thermals): 34.61,26.99 38.42,26.99 38.42,25.56 38.1,25.24 36.35,25.24
  pour Bottom (isolate 0.305): 0,80 0,8.26 44.45,8.26 44.45,12.06 49.53,12.06 49.53,20.95 62.23,20.95 62.23,71.12 65,71.12 65,80
INTRQ  (via drill 0.3)
  Top 0.203: XC1.31 15.24,75.56 v15.24,68.26 | v15.24,63.18 R4.2 16.03,62.07 17.46,60.64 18.41,60.64 19.39,59.67 IC7.5
  Bottom 0.203: v15.24,63.18 v15.24,68.26
M_INTRQ  (via drill 0.3)
  Top 0.152: IC1.36 19.87,28.28 17.46,25.88 12.86,25.88 10.32,28.42 10.32,32.54 12.86,35.08 v12.86,44.45 | IC7.3 18.74,53.66 12.86,47.78 v12.86,46.99
  Bottom 0.152: v12.86,46.99 v12.86,44.45
N$1
  Top 0.152: IC1.67 34.8,29.08 36.35,30.64 40.8,30.64 41.27,31.11 41.27,31.75 41.75,32.23 R6.2
N$2
  Top 0.152: IC1.66 34.87,28.68 36.51,30.32 R7.2
N$3
  Top 0.152: IC1.72 34.57,31.08 37.15,33.66 38.89,33.66 39.21,33.97 IC2.5
N$4
  Top 0.152: IC1.74 34.42,31.88 37.78,35.24 37.78,36.67 39.85,38.73 39.85,41.43 40.16,41.75 41.43,41.75 41.75,41.43 IC2.2
N$5
  Top 0.152: IC1.73 34.5,31.48 38.1,35.08 38.1,36.35 40.48,38.73 IC2.3
N$6
  Top 0.152: IC1.70 34.73,30.28 37.47,33.02 41.12,33.02 41.75,33.66 IC2.7
N$7
  Top 0.152: IC1.71 34.65,30.68 37.31,33.34 40.16,33.34 40.48,33.66 IC2.6
N$8
  Top 0.203: PB1.2 47.62,39.85 | PB1.1 47.62,39.37 47.62,39.85 | R15.2 47.62,39.85
N$9
  Top 0.152: IC1.75 34.34,32.28 37.47,35.4 37.47,38.26 38.1,38.89 38.1,41.59 | 43.02,41.75 IC2.1 | R14.1 37.94,41.75 38.1,41.59 | 43.02,41.75 R15.1 | 43.02,41.75 42.55,42.23 38.73,42.23 38.1,41.59
N$10
  Top 0.152: IC1.31 18.69,30.28 18.26,29.84 18.26,28.26 17.46,27.46 R13.1
N$11
  Top 0.203: R13.2 14.92,28.57 14.78,28.72 X1.1 13.49,29.68 13.34,29.53 C22.2
N$12
  Top 0.152: IC1.30 18.69,30.68 18.1,31.27 X1.3
  Top 0.203: X1.3 16.98,32.24 16.83,32.38 C23.2
N$13
  Top 0.203: IC1.63 35.86,27.48 35.88,27.46
  Top 0.406: 35.88,27.46 38.58,27.46 39.33,26.71 L1.1
N$14
  Top 0.406: IC9.1 39.37,20.64 37.48,18.75 USB.2
N$15
  Top 0.203: IC1.61 34.28,26.68 36.2,24.77 36.83,24.77 37.12,24.48 C19.2 37.12,23.05 37.31,22.86 R12.1
N$16
  Top 0.406: IC9.3 39.37,18.73 38.73,18.1 38.73,14.24 USB.3
N$17
  Top 0.152: RN6.1 45.03,52.18 45.4,52.55 45.4,54.88
  Top 0.203: 45.4,54.88 IC3.5
N$18
  Top 0.203: D3.A 19.68,15.24 19.05,15.88 19.05,18.41 18.41,19.05 R10.1
N$19
  Top 0.152: R9.2 16.51,22.86 15.88,22.23 15.88,16.19 15.4,15.72
  Top 0.203: D2.A 14.92,15.24 15.4,15.72 15.56,15.88
N$20
  Top 0.203: D4.A 26.04,15.24 25.4,15.88 25.4,18.41 24.77,19.05 R11.1
N$21
  Top 0.203: D1.A 6.99,15.24 6.35,15.88 6.35,18.41 5.71,19.05 R8.1
N$24
  Top 0.152: RN6.2 44.22,52.32 44.77,52.86 44.77,54.86
  Top 0.203: 44.77,54.86 IC3.4
N$25
  Top 0.152: RN6.3 43.41,52.62 44.09,53.3 IC3.3
N$26
  Top 0.152: IC3.2 43.45,53.76 42.6,52.91 RN6.4
N$27
  Top 0.152: IC3.9 47.99,53.76 48.84,52.91 RN7.1
N$28
  Top 0.152: RN7.2 48.03,52.62 47.34,53.3 IC3.8
N$29
  Top 0.152: RN7.3 47.22,52.32 46.67,52.86 46.67,54.86
  Top 0.203: 46.67,54.86 IC3.7
N$30
  Top 0.152: RN7.4 46.41,52.18 46.04,52.55 46.04,54.88
  Top 0.203: 46.04,54.88 IC3.6
N$31
  Top 0.152: RN8.1 34.56,52.18 34.92,52.55 IC4.5
  Top 0.203: IC4.5
N$32
  Top 0.152: RN8.2 33.74,52.32 34.29,52.86 34.29,54.86
  Top 0.203: 34.29,54.86 IC4.4
N$33
  Top 0.152: IC4.3 33.62,53.3 32.93,52.62 RN8.3
N$34
  Top 0.152: IC4.2 32.97,53.76 32.12,52.91 RN8.4
N$35
  Top 0.152: IC4.9 37.52,53.76 38.37,52.91 RN9.1
N$36
  Top 0.152: RN9.2 37.55,52.62 36.87,53.3 IC4.8
N$37
  Top 0.152: RN9.3 36.74,52.48 36.22,53 IC4.7
N$38
  Top 0.152: RN9.4 35.93,52.18 35.56,52.55 IC4.6
  Top 0.203: IC4.6
N$39
  Top 0.152: IC1.35 19.63,28.68 17.3,26.35 13.02,26.35 10.79,28.57 10.79,32.38 14.13,35.72 R16.1 14.92,36.51 14.38,37.06 PB2.1
  Top 0.203: PB2.1 PB2.2
N$40
  Top 1.27: SW1.1 59.95,11.05 57.78,8.89 49.53,8.89 45.09,4.45 33.02,4.45 26.71,10.75 PWR.1
N$41
  Top 1.27: SW1.4 62.87,16.77 62.87,10.16 59.05,6.35 50.8,6.35 46.35,1.91 17.1,1.91 PWR.4
OPT1_JMP
  Top 0.152: IC1.38 20.34,27.48 17.78,24.92 12.54,24.92 11.43,23.81 JP1.1
OPT2_JMP
  Top 0.152: IC1.39 20.57,27.08 17.94,24.45 14.61,24.45 13.97,23.81 JP2.1
PE
  Top 0.61: USB.S1 31.11,11.88 R17.2 | C26.2 46.35,11.88 USB.S2
  Bottom 1.778: SW1.S1 SW1.S2 45.6,10.28 USB.S2 USB.S1
USB_DM
  Top 0.406: R7.1 44.93,30.32 45.09,30.16 45.09,21.11 44.61,20.64 IC9.6
USB_DP
  Top 0.406: R6.1 45.09,32.23 45.72,31.59 45.72,19.68 44.77,18.73 IC9.4

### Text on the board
Top: BLASTER 2026
tPotisk: RESET | BOOT | IDE-USB BRIDGE | ACT | ERR | +5V | +12V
